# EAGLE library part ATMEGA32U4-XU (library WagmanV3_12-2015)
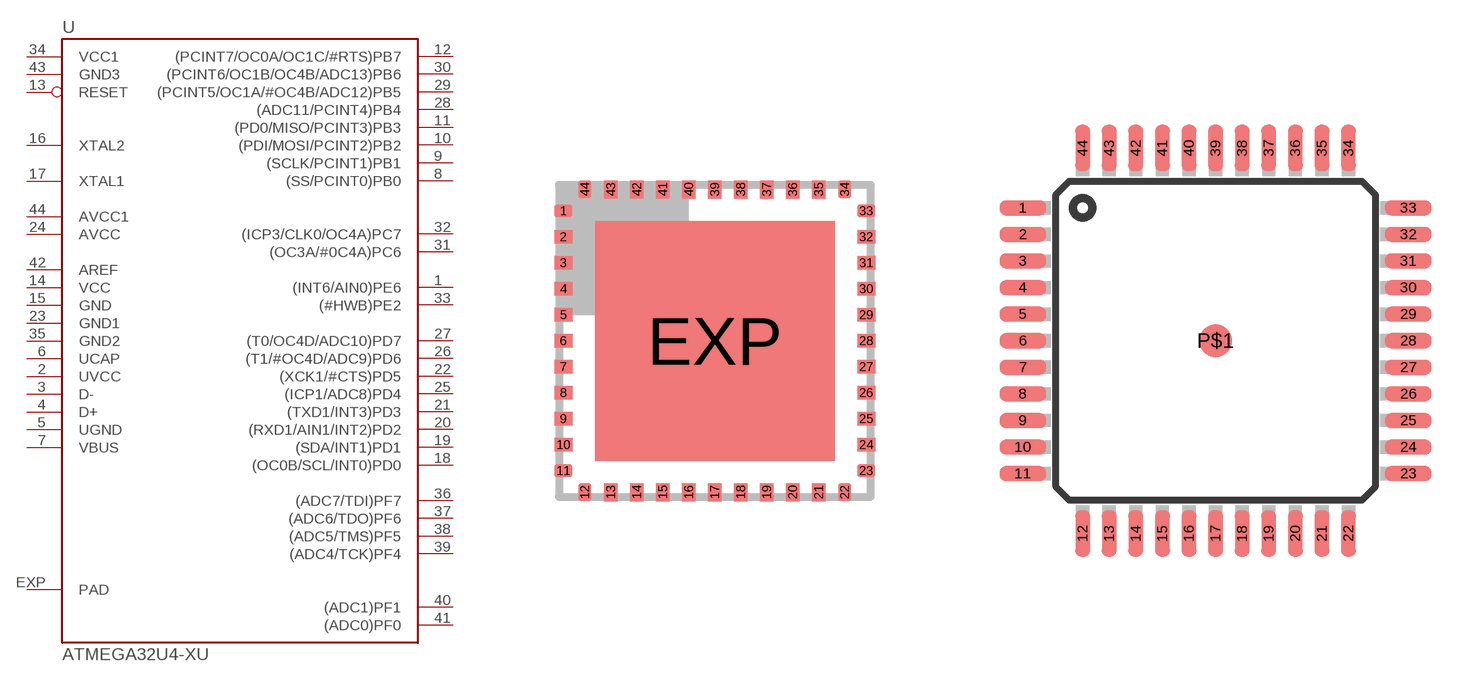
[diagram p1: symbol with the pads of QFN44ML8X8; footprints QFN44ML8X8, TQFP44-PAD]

Designator prefix -

## ATMEGA32U4-XU  [QFN44ML8X8]
1  (INT6/AIN0)PE6
2  UVCC  pwr
3  D-
4  D+
5  UGND  pwr
6  UCAP  pas
7  VBUS  in
8  (SS/PCINT0)PB0
9  (SCLK/PCINT1)PB1
10  (PDI/MOSI/PCINT2)PB2
11  (PD0/MISO/PCINT3)PB3
12  (PCINT7/OC0A/OC1C/#RTS)PB7
13  RESET  in
14  VCC  pwr
15  GND  pwr
16  XTAL2
17  XTAL1
18  (OC0B/SCL/INT0)PD0
19  (SDA/INT1)PD1
20  (RXD1/AIN1/INT2)PD2
21  (TXD1/INT3)PD3
22  (XCK1/#CTS)PD5
23  GND1  pwr
24  AVCC  pwr
25  (ICP1/ADC8)PD4
26  (T1/#OC4D/ADC9)PD6
27  (T0/OC4D/ADC10)PD7
28  (ADC11/PCINT4)PB4
29  (PCINT5/OC1A/#OC4B/ADC12)PB5
30  (PCINT6/OC1B/OC4B/ADC13)PB6
31  (OC3A/#0C4A)PC6
32  (ICP3/CLK0/OC4A)PC7
33  (#HWB)PE2
34  VCC1  pwr
35  GND2  pwr
36  (ADC7/TDI)PF7
37  (ADC6/TDO)PF6
38  (ADC5/TMS)PF5
39  (ADC4/TCK)PF4
40  (ADC1)PF1
41  (ADC0)PF0
42  AREF  pwr
43  GND3  pwr
44  AVCC1  pwr
EXP  PAD  pwr

## ATMEGA32U4-XUAU  [TQFP44-PAD]
1  (INT6/AIN0)PE6
2  UVCC  pwr
3  D-
4  D+
5  UGND  pwr
6  UCAP  pas
7  VBUS  in
8  (SS/PCINT0)PB0
9  (SCLK/PCINT1)PB1
10  (PDI/MOSI/PCINT2)PB2
11  (PD0/MISO/PCINT3)PB3
12  (PCINT7/OC0A/OC1C/#RTS)PB7
13  RESET  in
14  VCC  pwr
15  GND  pwr
16  XTAL2
17  XTAL1
18  (OC0B/SCL/INT0)PD0
19  (SDA/INT1)PD1
20  (RXD1/AIN1/INT2)PD2
21  (TXD1/INT3)PD3
22  (XCK1/#CTS)PD5
23  GND1  pwr
24  AVCC  pwr
25  (ICP1/ADC8)PD4
26  (T1/#OC4D/ADC9)PD6
27  (T0/OC4D/ADC10)PD7
28  (ADC11/PCINT4)PB4
29  (PCINT5/OC1A/#OC4B/ADC12)PB5
30  (PCINT6/OC1B/OC4B/ADC13)PB6
31  (OC3A/#0C4A)PC6
32  (ICP3/CLK0/OC4A)PC7
33  (#HWB)PE2
34  VCC1  pwr
35  GND2  pwr
36  (ADC7/TDI)PF7
37  (ADC6/TDO)PF6
38  (ADC5/TMS)PF5
39  (ADC4/TCK)PF4
40  (ADC1)PF1
41  (ADC0)PF0
42  AREF  pwr
43  GND3  pwr
44  AVCC1  pwr
P$1  PAD  pwr

## ATMEGA32U4-XUMU  [QFN44ML7X7]
Pads as for QFN44ML8X8

## Footprint QFN44ML8X8 (pad centres in mm)
44-Lead Plastic Quad Flat No Lead Package (ML) 8x8 mm Body (QFN) Source: http://ww1.microchip.com/downloads/en/devicedoc/39632c.pdf
smd 0.45 x 0.33: 1 -3.788,3.25; 2 -3.788,2.6; 3 -3.788,1.95; 4 -3.788,1.3; 5 -3.788,0.65; 6 -3.788,0; 7 -3.788,-0.65; 8 -3.788,-1.3; 9 -3.788,-1.95; 10 -3.788,-2.6; 11 -3.788,-3.25; 23 3.788,-3.25; 24 3.788,-2.6; 25 3.788,-1.95; 26 3.788,-1.3; 27 3.788,-0.65; 28 3.788,0; 29 3.788,0.65; 30 3.788,1.3; 31 3.788,1.95; 32 3.788,2.6; 33 3.788,3.25
smd 0.33 x 0.45: 12 -3.25,-3.788; 13 -2.6,-3.788; 14 -1.95,-3.788; 15 -1.3,-3.788; 16 -0.65,-3.788; 17 0,-3.788; 18 0.65,-3.788; 19 1.3,-3.788; 20 1.95,-3.788; 21 2.6,-3.788; 22 3.25,-3.788; 34 3.25,3.788; 35 2.6,3.788; 36 1.95,3.788; 37 1.3,3.788; 38 0.65,3.788; 39 0,3.788; 40 -0.65,3.788; 41 -1.3,3.788; 42 -1.95,3.788; 43 -2.6,3.788; 44 -3.25,3.788
smd 6 x 6: EXP 0,0

## Footprint TQFP44-PAD (pad centres in mm)
44-lead Thin Quad Flat Package
smd 1.4 x 0.45: 1 -5.8,4; 2 -5.8,3.2; 3 -5.8,2.4; 4 -5.8,1.6; 5 -5.8,0.8; 6 -5.8,0; 7 -5.8,-0.8; 8 -5.8,-1.6; 9 -5.8,-2.4; 10 -5.8,-3.2; 11 -5.8,-4; 23 5.8,-4; 24 5.8,-3.2; 25 5.8,-2.4; 26 5.8,-1.6; 27 5.8,-0.8; 28 5.8,0; 29 5.8,0.8; 30 5.8,1.6; 31 5.8,2.4; 32 5.8,3.2; 33 5.8,4
smd 0.45 x 1.4: 12 -4,-5.8; 13 -3.2,-5.8; 14 -2.4,-5.8; 15 -1.6,-5.8; 16 -0.8,-5.8; 17 0,-5.8; 18 0.8,-5.8; 19 1.6,-5.8; 20 2.4,-5.8; 21 3.2,-5.8; 22 4,-5.8; 34 4,5.8; 35 3.2,5.8; 36 2.4,5.8; 37 1.6,5.8; 38 0.8,5.8; 39 0,5.8; 40 -0.8,5.8; 41 -1.6,5.8; 42 -2.4,5.8; 43 -3.2,5.8; 44 -4,5.8
smd 1 x 1: P$1 0,0

## Footprint QFN44ML7X7 (pad centres in mm)
smd 0.75 x 0.275: 1 -3.275,2.5; 2 -3.275,2; 3 -3.275,1.5; 4 -3.275,1; 5 -3.275,0.5; 6 -3.275,0; 7 -3.275,-0.5; 8 -3.275,-1; 9 -3.275,-1.5; 10 -3.275,-2; 11 -3.275,-2.5; 23 3.275,-2.5; 24 3.275,-2; 25 3.275,-1.5; 26 3.275,-1; 27 3.275,-0.5; 28 3.275,0; 29 3.275,0.5; 30 3.275,1; 31 3.275,1.5; 32 3.275,2; 33 3.275,2.5
smd 0.275 x 0.75: 12 -2.5,-3.275; 13 -2,-3.275; 14 -1.5,-3.275; 15 -1,-3.275; 16 -0.5,-3.275; 17 0,-3.275; 18 0.5,-3.275; 19 1,-3.275; 20 1.5,-3.275; 21 2,-3.275; 22 2.5,-3.275; 34 2.5,3.275; 35 2,3.275; 36 1.5,3.275; 37 1,3.275; 38 0.5,3.275; 39 0,3.275; 40 -0.5,3.275; 41 -1,3.275; 42 -1.5,3.275; 43 -2,3.275; 44 -2.5,3.275
smd 4.826 x 4.826: EXP 0,0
